PROGRAM MAIN_CM
VAR CONSTANT
	cInitSpectrum 	: ST_CM_MagnitudeSpectrum_InitPars 	:= (	nFFT_Length 		:= cFFTLength, 
																nWindowLength 		:= cWindowLength, 
																bTransformToDecibel	:= TRUE, 
																eWindowType 		:= E_CM_WindowType.eCM_HannWindow, 
																eScalingType 		:= E_CM_ScalingType.eCM_PowerSpectralDensity,
																nChannels			:= cChannels);
															
	cInitStatistics	: ST_CM_WindowStatistics_InitPars 	:= ( 	nInLength			:= cFFTResult,
																nMaxWindows			:= cMaxWindows,
																nChannels			:= cChannels,
																fScaleFactor		:= cSampleRate/cFFTLength);
END_VAR
VAR	
	fbSpectrum			: FB_CMA_MagnitudeSpectrum := (stInitPars := cInitSpectrum, nOwnID := eID_Spectrum, aDestIDs := [eID_SinkSpectrum, eID_Statistics]);
	fbWindowStatistics	: FB_CMA_WindowStatistics := (stInitPars := cInitStatistics, nOwnID := eID_Statistics, aDestIDs := [eID_SinkStatistics]);
	
	nWindow				: UDINT;
	aConfigArgs			: ARRAY[1..cMaxWindows] OF ARRAY[1..2] OF LREAL;  // window limits, i.e. lower and upper bounds
	fDiameter			: LREAL := 200.0;
	
	bConfigure			: BOOL := TRUE;
	fbErrHist			: FB_HRErrHist; // error monitoring
END_VAR

IF bConfigure THEN
	// Set limits
	FOR nWindow := 1 TO cMaxWindows DO
		aConfigArgs[nWindow][1] := MAX(MAIN.aSetFrequency[1][nWindow] - fDiameter/2,0);
		aConfigArgs[nWindow][2] := MAX(MAIN.aSetFrequency[1][nWindow] + fDiameter/2,0);
	END_FOR
	
	// Configure window statistics
	fbWindowStatistics.Configure(ADR(aConfigArgs), SIZEOF(aConfigArgs));
	IF fbWindowStatistics.bError THEN
		fbErrHist.AddError(bErr:=TRUE, hrErrCode:=fbWindowStatistics.hrErrorCode, sErrSource:='MAIN_CM.fbWindowStatistics.Configure'); // error monitoring
		// ToDo: if error
	ELSE
		bConfigure := FALSE;
	END_IF
END_IF

// Call spectrum call
fbSpectrum.Call();
IF fbSpectrum.bError THEN
	fbErrHist.AddError(bErr:=TRUE, hrErrCode:=fbSpectrum.hrErrorCode, sErrSource:='MAIN_CM.fbSpectrum.Call'); // error monitoring
	// ToDo: if error
END_IF

// Call window statistics call
fbWindowStatistics.Call();
IF fbWindowStatistics.bError THEN
	fbErrHist.AddError(bErr:=TRUE, hrErrCode:=fbWindowStatistics.hrErrorCode, sErrSource:='MAIN_CM.fbWindowStatistics.Call'); // error monitoring
	// ToDo: if error
END_IF

END_PROGRAM
